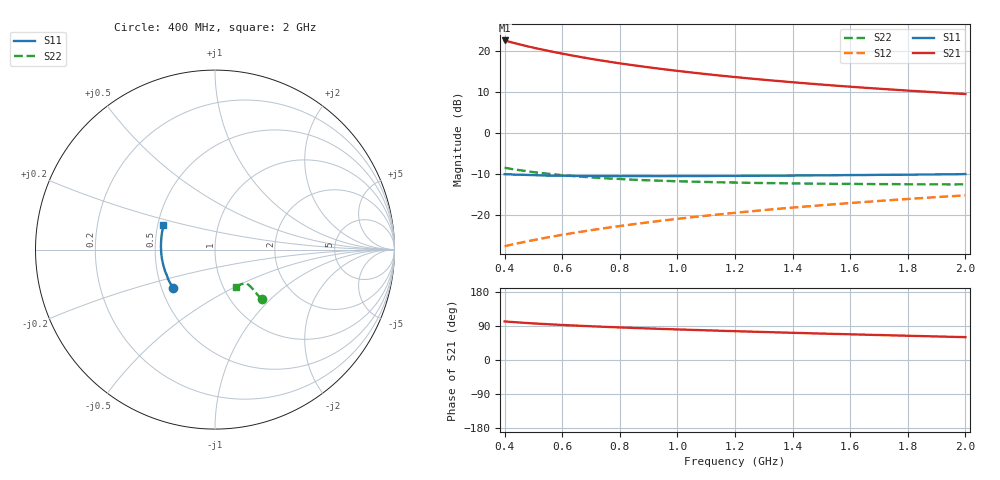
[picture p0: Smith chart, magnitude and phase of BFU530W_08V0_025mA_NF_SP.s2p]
! Filename:  P:\Prog\Test\Noise\ATS_data\Testdata_Net\06 Compressed Noise after Statistics\BFU530W_APM2013_09_A05_08p0V_025mA_NF_CM01_D.sf
! Date/Time: Tue 26/Mar/2013 18:06:02
! BFU530W_APM2013_09_A05_08p0V_1to25mA_NF_CM01_Bias9_R.sf
! Noise Parameter Data File
! BFU530W_APM2013_09_A05_08p0V_1to25mA_NF_CM01
! Date/time: Thu Mar 21 21:44:48 2013
! VAR V_out= 8.000000
! VAR I_out= 25.005000
! VAR V_in= 0.801300
! VAR I_in= 0.253100
! Device data file deembeded for feedlines and parallel
! Original file: \06 Compressed Noise after Statistics\BFU530W_APM2013_09_A05_08p0V_025mA_NF_CM01_R.sf
! Feed-files: PR019V01_070313_Feed1.s2p, PR019V01_070313_Feed2.s2p
! Parallel-file: PR019V01_070313_Par.s2p
# MHz S MA R 50
!  Freq-MHz  S11-mag  S11-arg  S21-mag  S21-arg  S12-mag  S12-arg  S22-mag  S22-arg
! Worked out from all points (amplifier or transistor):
!   37 points, 400 MHz to 2 GHz, reference 50 ohm
!   highest |S21| = 22.6 dB at 400 MHz (marker M1)
!   |S21| within 3 dB of that: start of sweep to 584.5 MHz
!   unconditionally stable (mu >= 1): 990.7 MHz to end of sweep
!   at 500 MHz: K = 0.90, MSG = 23.5 dB, |S12| = -26.1 dB
!   at 1.1 GHz: K = 1.01, MAG = 16.8 dB, |S12| = -20.1 dB
!   at 2 GHz: K = 1.01, MAG = 11.8 dB, |S12| = -15.2 dB
!   lowest NFmin = 1.12 dB at 420 MHz
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400  0.3166 -137.2  13.56 101.8  0.04188 67.5  0.3791 -46.7
420  0.315 -139.8  12.98 100.6  0.04343 67.7  0.3687 -46.8
440  0.3127 -142.0  12.45 99.5  0.04495 68.1  0.359 -46.8
460  0.3114 -144.0  11.95 98.5  0.04652 68.4  0.351 -46.8
480  0.3099 -146.1  11.5 97.5  0.04807 68.6  0.3431 -46.7
500  0.3084 -148.0  11.07 96.6  0.04959 68.9  0.3353 -46.6
550  0.3038 -152.1  10.15 94.4  0.05362 69.5  0.3206 -46.4
600  0.3034 -155.9  9.364 92.5  0.05758 70.0  0.3075 -46.2
650  0.3017 -159.4  8.685 90.7  0.06156 70.3  0.2978 -46.2
700  0.3008 -162.5  8.097 89.0  0.06563 70.7  0.2894 -46.2
750  0.3004 -165.2  7.584 87.5  0.06966 70.9  0.2819 -46.1
800  0.2998 -168.0  7.133 86.0  0.07376 71.1  0.2767 -46.4
850  0.3002 -170.5  6.734 84.6  0.07783 71.2  0.2707 -46.4
950  0.2996 -174.8  6.058 81.9  0.08612 71.5  0.263 -46.9
1050  0.3005 -178.7  5.507 79.5  0.09441 71.5  0.257 -47.6
1150  0.3016 177.6  5.048 77.2  0.1027 71.3  0.2516 -48.4
1200  0.3016 176.0  4.851 76.0  0.107 71.2  0.2504 -49.1
1350  0.3035 171.4  4.34 72.8  0.1196 70.8  0.2459 -50.7
1500  0.3063 167.0  3.928 69.7  0.1322 70.2  0.2426 -53.0
1650  0.3091 163.0  3.592 66.9  0.1449 69.5  0.2402 -55.1
1750  0.3112 160.7  3.405 64.9  0.1535 69.0  0.2396 -56.6
2000  0.3175 154.8  3.01 60.3  0.1746 67.5  0.2381 -61.2
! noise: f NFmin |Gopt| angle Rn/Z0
400  1.143  0.281  -171.7  0.0829
460  1.16  0.2887  -171.2  0.0795
600  1.176  0.2892  -168  0.0817
800  1.199  0.3015  -164.4  0.0821
1000  1.218  0.3137  -160.2  0.0819
1200  1.27  0.3178  -157.2  0.0854
1400  1.295  0.3224  -153.7  0.0897
1600  1.293  0.3305  -149.3  0.0968
1800  1.32  0.3559  -146.3  0.0958
2000  1.367  0.3711  -142.8  0.0987
